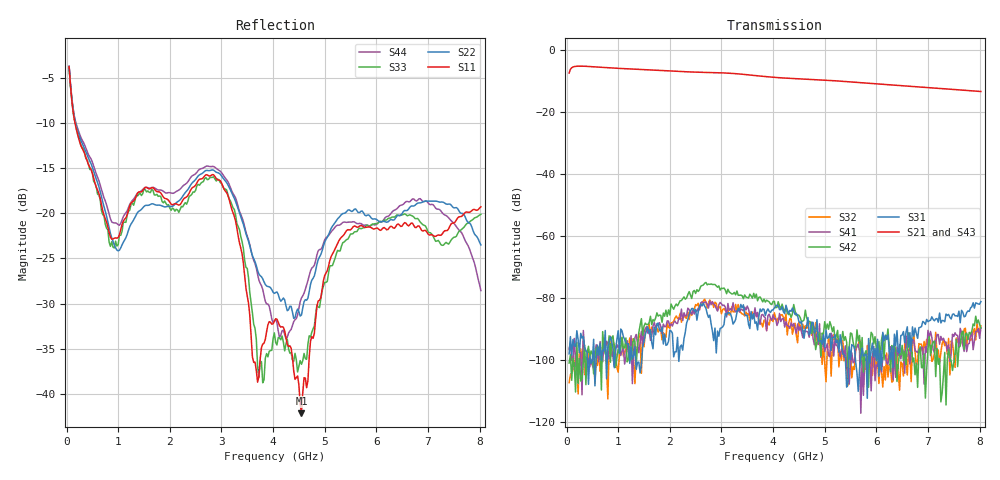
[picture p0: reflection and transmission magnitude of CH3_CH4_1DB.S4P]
!Agilent Technologies,E5071C,MY46316741,A.11.02
!Date: Thu May 28 15:04:23 2026
!Data & Calibration Information:
!1:CH3 INPUT 2:CH3 OUTPUT 3:CH4 INPUT 4:CH4 OUTPUT
!Freq	S11:SOLT4(ON)	S12:SOLT4(ON)	S13:SOLT4(ON)	S14:SOLT4(ON)
!	S21:SOLT4(ON)	S22:SOLT4(ON)	S23:SOLT4(ON)	S24:SOLT4(ON)
!	S31:SOLT4(ON)	S32:SOLT4(ON)	S33:SOLT4(ON)	S34:SOLT4(ON)
!	S41:SOLT4(ON)	S42:SOLT4(ON)	S43:SOLT4(ON)	S44:SOLT4(ON)
!PortZ  Port1:50+j0  Port2:50+j0  Port3:50+j0  Port4:50+j0
!Above PortZ is port z conversion or system Z0 setting when saving the data.
!When reading, reference impedance value at option line is always used.
# Hz S dB R 50
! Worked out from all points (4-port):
!   320 points, 50 MHz to 8.025 GHz, reference 50 ohm
!   strongest paths, dB at 50 MHz, 2.05 GHz, 4.05 GHz, 6.05 GHz, 8.025 GHz:
!     S21: -7.4, -6.8, -8.8, -11.0, -13.4
!     S43: -7.4, -6.8, -8.9, -11.1, -13.5
!     S31: -98.0, -91.2, -82.6, -105.2, -81.1
!     S42: -100.9, -82.9, -83.1, -94.0, -89.6
!     S41: -96.5, -89.0, -86.5, -98.1, -89.5
!     S32: -107.3, -88.0, -86.4, -107.5, -88.9
!   lowest |S11| = -42.1 dB at 4.55 GHz (marker M1), VSWR 1.02, Z = 49.6 - j0.66 ohm
!   |S11| at or under -10 dB: 164 MHz to end of sweep
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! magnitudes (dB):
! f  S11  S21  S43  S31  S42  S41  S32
! 50 MHz  -3.8  -7.4  -7.4  -98.0  -100.9  -96.5  -107.3
! 975 MHz  -22.8  -5.9  -5.9  -93.4  -99.2  -95.0  -102.4
! 2.975 GHz  -16.4  -7.3  -7.4  -89.8  -77.4  -81.4  -82.7
! 3.725 GHz  -38.1  -8.3  -8.4  -85.8  -79.7  -87.6  -86.8
! 4.55 GHz  -42.1  -9.3  -9.4  -87.5  -87.5  -90.8  -90.7
! 5.425 GHz  -21.9  -10.2  -10.2  -108.7  -94.2  -101.6  -102.1
! 8.025 GHz  -19.3  -13.4  -13.5  -81.1  -89.6  -89.5  -88.9
